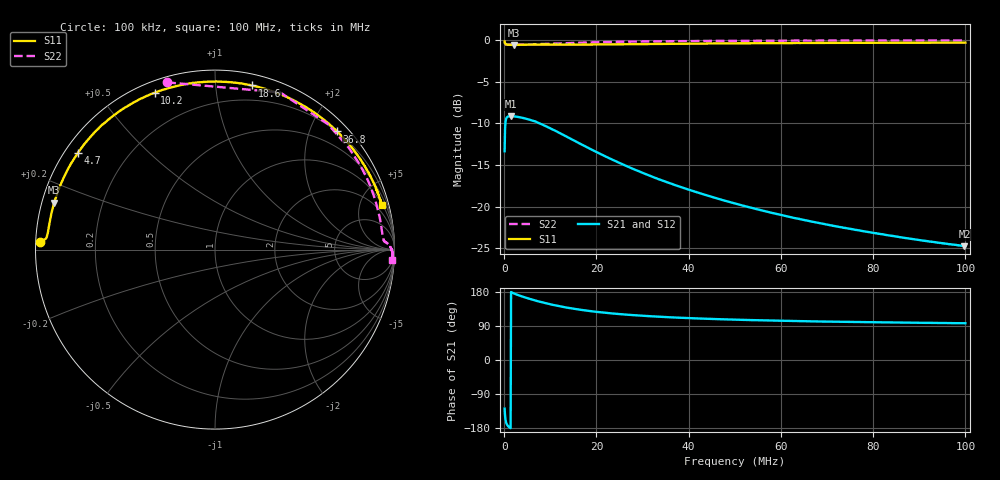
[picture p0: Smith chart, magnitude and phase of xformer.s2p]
# Hz S RI R 50.0
! written by SimSmith version 18.3h
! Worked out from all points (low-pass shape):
!   1000 points, 100 kHz to 100 MHz, reference 50 ohm
!   highest |S21| = -9.15 dB at 1.5 MHz (marker M1); lowest = -24.7 dB at 99.8 MHz (marker M2)
!   |S21| within 3 dB of the highest: 144.3 kHz to 15.43 MHz (15.29 MHz wide, 196 % of centre)
!   lowest |S11| = -0.6 dB at 2.1 MHz (marker M3), VSWR 28.65, Z = 1.78 + j7.15 ohm
!   |S11| at or under -10 dB: nowhere
!   |S22| runs from -0.6 to -0.1 dB; largest |S21 - S12| = 0.0015
!   S11 on the Smith chart (normalised r, x): 100 kHz: 0.01, +0.02; 4.7 MHz: 0.04, +0.32; 10.2 MHz: 0.05, +0.69; 18.6 MHz: 0.08, +1.25; 36.8 MHz: 0.19, +2.46; 100 MHz: 1.09, +7.40
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100000  -0.9767 0.0403  -0.1332 -0.1686  -0.1343 -0.1691  -0.2663 0.9317
700000  -0.9302 0.0997  -0.3419 -0.0475  -0.3424 -0.0471  0.8682 0.3475
800000  -0.9284 0.1107  -0.3444 -0.0374  -0.345 -0.0374  0.8822 0.3067
1000000  -0.9249 0.1334  -0.3472 -0.0222  -0.3476 -0.0222  0.9004 0.249
1500000  -0.9133 0.1918  -0.3488 0.00394  -0.349 0.00411  0.9195 0.17
2100000  -0.8951 0.2617  -0.3468 0.026  -0.3474 0.0262  0.927 0.1252
3100000  -0.8552 0.3744  -0.3404 0.0545  -0.3408 0.0544  0.932 0.0893
4700000  -0.7648 0.5376  -0.3247 0.0905  -0.3251 0.0904  0.937 0.0649
7400000  -0.564 0.7481  -0.2879 0.1354  -0.2886 0.1354  0.9416 0.0494
1.02e7  -0.3355 0.8743  -0.2442 0.1619  -0.245 0.1619  0.9466 0.0433
1.31e7  -0.1164 0.9289  -0.2023 0.174  -0.2031 0.1739  0.9532 0.0392
1.68e7  0.1141 0.9297  -0.1581 0.1753  -0.1589 0.1754  0.961 0.0346
1.86e7  0.2054 0.9144  -0.1406 0.1723  -0.1414 0.1727  0.9645 0.0322
2.16e7  0.3339 0.8772  -0.116 0.1658  -0.1168 0.1662  0.9686 0.0273
2.52e7  0.4529 0.8241  -0.0937 0.1559  -0.0941 0.1563  0.9735 0.0219
3.34e7  0.6313 0.7041  -0.0606 0.1334  -0.0608 0.1341  0.9794 0.01
3.68e7  0.6804 0.6586  -0.0513 0.1255  -0.0516 0.126  0.9815 0.00639
5.01e7  0.8009 0.5164  -0.0295 0.1002  -0.0297 0.1007  0.9863 -0.00948
6.67e7  0.8721 0.3955  -0.017 0.0796  -0.0171 0.0801  0.989 -0.0266
8.34e7  0.9082 0.3122  -0.0108 0.0665  -0.0108 0.0669  0.99 -0.043
9.98e7  0.9288 0.251  -0.00722 0.0576  -0.00714 0.058  0.9883 -0.0594
1e8  0.9291 0.2503  -0.0071 0.0576  -0.00709 0.0579  0.9888 -0.0601
